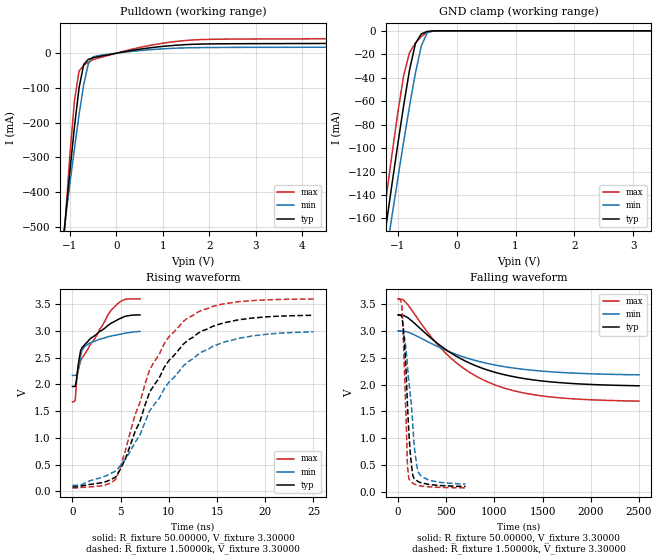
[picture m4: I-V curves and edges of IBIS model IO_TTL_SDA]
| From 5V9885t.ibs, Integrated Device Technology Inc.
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|   Model IO_TTL_SDA
[Model]   IO_TTL_SDA
Model_type   I/O_open_sink
Polarity   Non-Inverting
Vinl =  0.80000V
Vinh =  2.00000V
Vmeas =  1.65000V
C_comp   3.90000pF   3.90000pF   3.90000pF
[Temperature Range]   25.00000   100.00000   -40.00000
[Voltage Range]   3.30000V   3.00000V   3.60000V
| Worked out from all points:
|   slope of the pulldown table from 0 to 0.495 V, typ, clamps not added: 43.5 ohm
|   GND clamp passes 1 mA (typ) near -0.52 V on its own axis
|   rising waveform, R_fixture 50.00000, V_fixture 3.30000: 20-80 % time 2.7ns typ, 1.89ns min, 3.01ns max; typ from 1.96 V to 3.3 V
|   rising waveform, R_fixture 1.50000k, V_fixture 3.30000: 20-80 % time 5.32ns typ, 6.11ns min, 4.5ns max; typ from 0.084 V to 3.29 V
|   falling waveform, R_fixture 50.00000, V_fixture 3.30000: 20-80 % time 745ns typ, 797ns min, 692ns max; typ from 3.3 V to 1.98 V
|   falling waveform, R_fixture 1.50000k, V_fixture 3.30000: 20-80 % time 55.4ns typ, 83.7ns min, 39.4ns max; typ from 3.3 V to 0.098 V
[Pulldown]
| voltage   I(typ)   I(min)   I(max)
-3.3V     -3.766A    -2.968A    -5.052A
-1.3V     -769.4mA   -703.4mA   -881.9mA
-1V       -344.3mA   -379.3mA   -298.9mA
-900mV    -213.2mA   -275.9mA   -138.2mA
-800mV    -100.1mA   -177.7mA   -51.19mA
-700mV    -32.56mA   -90.56mA   -35.2mA
-600mV    -17.75mA   -30.02mA   -25.79mA
-500mV    -13.24mA   -10.47mA   -18.79mA
600mV     13.4mA     8.771mA    19.31mA
1.5V      24.87mA    15.54mA    36.84mA
5.1V      29.24mA    17.99mA    43.76mA
6.6V      42.47mA    25.45mA    67.13mA
[GND_clamp]
| voltage   I(typ)   I(min)   I(max)
-3.3V     -941mA     -907.6mA   -976.3mA
-1.3V     -202.4mA   -224.6mA   -181.6mA
-1.2V     -166.7mA   -191.4mA   -143.4mA
-1.1V     -131.5mA   -158.6mA   -106mA
-1V       -96.95mA   -126.3mA   -70.13mA
-900mV    -63.73mA   -94.63mA   -38.18mA
-800mV    -33.34mA   -64.12mA   -18.46mA
-700mV    -10.74mA   -35.84mA   -10.48mA
-600mV    -2.575mA   -12.79mA   -4.779mA
-500mV    -539.2uA   -1.691mA   -1.235mA
-400mV    -63.38uA   -109.7uA   -138.9uA
3.3V      1.086nA    4.119nA    592.1pA
[Ramp]
| variable   typ   min   max
dV/dt_r   1.92508/5.19520n   1.72182/6.10290n   2.11914/4.49638n
dV/dt_f   1.92147/55.29974n   1.71552/81.65226n   2.11722/40.58984n
R_load = 1.50000k
[Rising Waveform]
R_fixture = 50.00000
V_fixture = 3.30000
V_fixture_min = 3.00000
V_fixture_max = 3.60000
| time   V(typ)   V(min)   V(max)
0s        1.96V      2.167V     1.674V
280ps     1.961V     2.167V     1.703V
420ps     2.099V     2.171V     2.041V
560ps     2.318V     2.227V     2.253V
840ps     2.628V     2.535V     2.442V
980ps     2.685V     2.632V     2.491V
1.82ns    2.849V     2.774V     2.737V
3.78ns    3.115V     2.894V     3.327V
5.32ns    3.262V     2.952V     3.581V
7ns       3.299V     2.991V     3.599V
[Rising Waveform]
R_fixture = 1.50000k
V_fixture = 3.30000
V_fixture_min = 3.00000
V_fixture_max = 3.60000
| time   V(typ)   V(min)   V(max)
0s        83.54mV    113.3mV    64.1mV
4.5ns     268.8mV    380.5mV    223.7mV
5.5ns     615.4mV    601.9mV    769mV
6.5ns     1.121V     917.6mV    1.436V
7ns       1.309V     1.054V     1.66V
8ns       1.855V     1.503V     2.273V
10ns      2.446V     2.04V      2.89V
11.5ns    2.752V     2.344V     3.177V
16ns      3.163V     2.804V     3.515V
25ns      3.292V     2.982V     3.596V
[Falling Waveform]
R_fixture = 50.00000
V_fixture = 3.30000
V_fixture_min = 3.00000
V_fixture_max = 3.60000
| time   V(typ)   V(min)   V(max)
0s        3.3V       3V         3.6V
50ns      3.296V     2.998V     3.587V
100ns     3.251V     2.982V     3.494V
350ns     2.855V     2.763V     2.874V
550ns     2.588V     2.6V       2.49V
750ns     2.394V     2.475V     2.219V
950ns     2.259V     2.385V     2.034V
1.2us     2.147V     2.308V     1.885V
1.5us     2.066V     2.25V      1.786V
2.5us     1.976V     2.181V     1.69V
[Falling Waveform]
R_fixture = 1.50000k
V_fixture = 3.30000
V_fixture_min = 3.00000
V_fixture_max = 3.60000
| time   V(typ)   V(min)   V(max)
0s        3.3V       3V         3.6V
42ns      3.262V     2.996V     3.442V
70ns      2.688V     2.847V     2.087V
98ns      1.611V     2.341V     473.4mV
112ns     1.111V     2.056V     243.5mV
140ns     485.4mV    1.603V     179.4mV
154ns     296mV      1.221V     155.3mV
168ns     242.8mV    847.9mV    138.9mV
210ns     186.7mV    363.7mV    115.8mV
700ns     97.55mV    140.8mV    71.3mV
